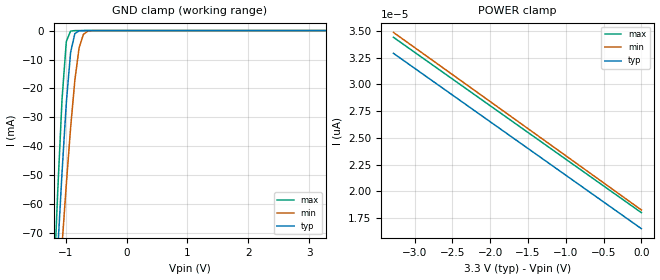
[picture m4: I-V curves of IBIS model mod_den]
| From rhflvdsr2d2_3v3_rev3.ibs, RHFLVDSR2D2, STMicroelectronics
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|   Model mod_den
[Model]   mod_den
Model_type Input
Vinl   =   0.8000V
Vinh   =   2.0000V
C_comp   0.085pF   0.082pF   0.088pF
[Temperature Range]  25.0000   0.1250k   -55.0000
[Voltage Range]   3.3000V   3.0000V   3.6000V
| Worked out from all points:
|   GND clamp passes 1 mA (typ) near -0.85 V on its own axis
[GND_clamp]
|Voltage   I(typ)   I(min)   I(max)
-3.3V     -1.037A    -847.3mA   -1.291A
-1.2V     -103.9mA   -118.4mA   -90.61mA
-1.13V    -75.7mA    -95.97mA   -55.15mA
-1.06V    -48.91mA   -74.09mA   -23.64mA
-990mV    -24.98mA   -53.14mA   -3.767mA
-920mV    -7.584mA   -33.75mA   -179uA
-850mV    -1.056mA   -17.22mA   -4.994uA
-780mV    -96.57uA   -5.968mA   -121.2nA
-710mV    -6.743uA   -1.337mA   -2.93nA
-640mV    -444.3nA   -233uA     -73.86pA
-500mV    -1.914nA   -4.408uA   -2.541pA
3.28V     16.4pA     19.67pA    16.4pA
[POWER_clamp]
|Voltage   I(typ)   I(min)   I(max)
-3.28V    32.9pA     34.86pA    34.4pA
-2.44V    28.7pA     30.61pA    30.2pA
-1.4V     23.5pA     25.35pA    25pA
0V        16.5pA     18.25pA    18pA
